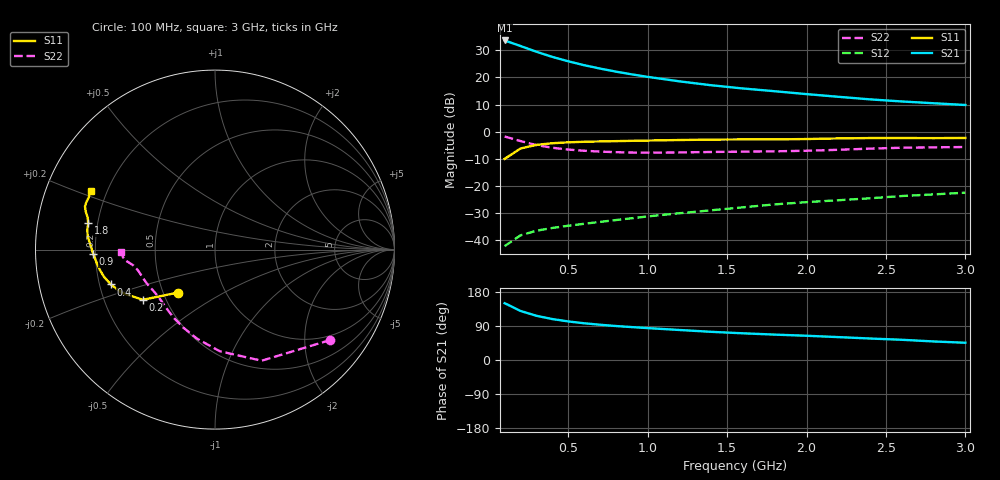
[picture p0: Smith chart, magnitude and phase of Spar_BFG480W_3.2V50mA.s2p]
! Filename: 3_250BFG480.001
! Title: BFG480W
! Bias: Vce=3.2V; Ic=50mA
! Company: NXP Semiconductors NL
! User: Quality&Reliability T&D
! Measure time: 10 Nov 1999 / 11:56:58
#  MHz  S  MA  R 50
! Freq  S11  S21  S12  S22  :
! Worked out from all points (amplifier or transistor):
!   20 points, 100 MHz to 3 GHz, reference 50 ohm
!   highest |S21| = 33.6 dB at 100 MHz (marker M1)
!   |S21| within 3 dB of that: start of sweep to 245.4 MHz
!   unconditionally stable (mu >= 1): 956.3 MHz to end of sweep
!   at 400 MHz: K = 0.64, MSG = 31.5 dB, |S12| = -35.5 dB
!   at 1.2 GHz: K = 1.05, MAG = 22.9 dB, |S12| = -30.0 dB
!   at 3 GHz: K = 1.07, MAG = 14.6 dB, |S12| = -22.5 dB
!   S11 on the Smith chart (normalised r, x): 100 MHz: 0.60, -0.32; 200 MHz: 0.37, -0.27; 400 MHz: 0.25, -0.15; 900 MHz: 0.19, -0.02; 1.8 GHz: 0.16, +0.10; 3 GHz: 0.14, +0.22
100  0.3155 -130.7  47.83 149.9  0.00779 68.1  0.8162 -38.1
200  0.49 -145.2  37.83 129.5  0.01233 56.8  0.6714 -67.2
300  0.5709 -155.0  29.64 116.7  0.015 52.9  0.5671 -87.3
400  0.6122 -161.5  23.84 108.1  0.01685 52.7  0.5055 -101.6
500  0.6364 -166.2  19.78 101.8  0.01852 53.8  0.4685 -112.3
600  0.6513 -169.9  16.78 96.9  0.02012 55.5  0.4454 -120.5
700  0.6615 -172.9  14.54 93.0  0.02179 57.6  0.4299 -126.9
800  0.6695 -175.6  12.77 89.7  0.02358 59.6  0.4193 -132.2
900  0.6784 -177.9  11.36 86.9  0.02546 61.7  0.4131 -136.8
1000  0.6861 180.0  10.22 84.2  0.02748 63.3  0.4106 -140.9
1200  0.702 176.3  8.449 79.2  0.03147 65.9  0.4145 -147.7
1400  0.7142 173.7  7.161 74.4  0.03565 67.8  0.4229 -152.8
1600  0.7201 171.1  6.246 70.4  0.04045 69.5  0.4286 -156.7
1800  0.7212 168.3  5.555 67.0  0.04583 70.9  0.4348 -160.6
2000  0.7319 165.8  4.917 64.0  0.0504 72.0  0.4452 -165.2
2200  0.7515 163.5  4.39 60.4  0.05464 72.5  0.4637 -169.1
2400  0.7635 161.6  3.935 56.7  0.05936 72.4  0.4875 -171.7
2600  0.7642 159.9  3.599 53.4  0.06529 72.1  0.506 -173.4
2800  0.7612 157.6  3.338 48.9  0.06997 71.1  0.5148 -175.4
3000  0.7661 154.9  3.099 45.5  0.07525 70.5  0.5222 -178.4
